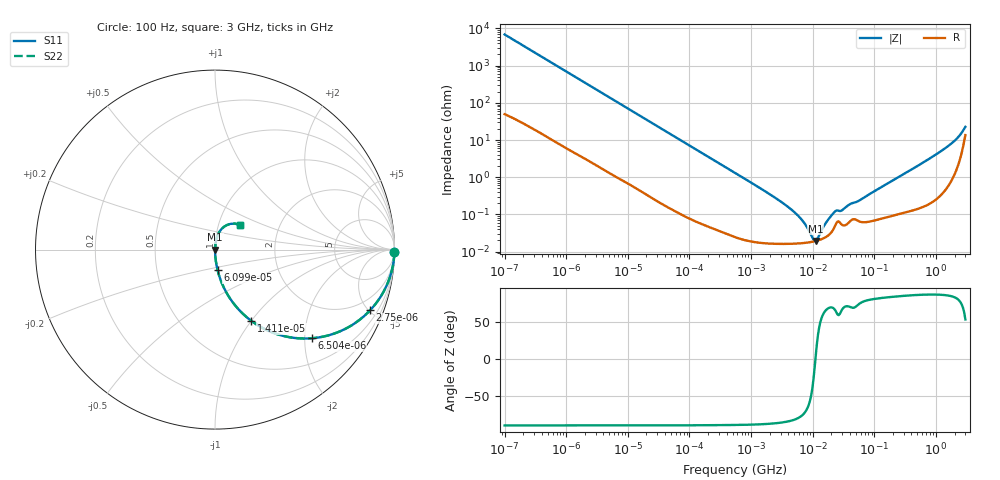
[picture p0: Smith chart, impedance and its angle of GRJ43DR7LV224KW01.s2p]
!Murata Part Number: GRJ43DR7LV224KW01
!These Parameters are Measured in Series Mode Connection
!Data Generated on Jun 19, 2026
!  o--ll--o
!Port1  Port2
!  o------o
!Operation Temp=25[degC], DC Bias Voltage=0[V]
!Freq. Start=100[Hz] Stop=3[GHz] 401[Steps]
# Hz S RI R 50
!Freq.(Hz) S11(Real) S11(Imag) S21(Real) S21(Imag) S12(Real) S12(Imag) S22(Real) S22(Imag)
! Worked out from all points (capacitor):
!   401 points, 100 Hz to 3 GHz, reference 50 ohm
!   read as one part in series: C = 232 nF near 109 Hz
!   lowest |Z| = 19.3 mohm at 11.14 MHz (marker M1)
!   series resonance near 11.06 MHz, so ESL is about 890 pH
!   S11 on the Smith chart (normalised r, x): 100 Hz: open; 2.75 kHz: 1.05, -5.08; 6.504 kHz: 1.02, -2.16; 14.12 kHz: 1.01, -1.00; 60.99 kHz: 1.00, -0.23; 3 GHz: 1.27, +0.36
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100  0.9997 -0.0146  0.000317 0.0146  0.000317 0.0146  0.9997 -0.0146
536  0.9934 -0.0768  0.00659 0.0768  0.00659 0.0768  0.9934 -0.0768
1788  0.9364 -0.2396  0.0636 0.2396  0.0636 0.2396  0.9364 -0.2396
2750  0.8637 -0.3385  0.1363 0.3385  0.1363 0.3385  0.8637 -0.3385
6504  0.5381 -0.4939  0.4619 0.4939  0.4619 0.4939  0.5381 -0.4939
14115  0.2024 -0.397  0.7976 0.397  0.7976 0.397  0.2024 -0.397
31977  0.0487 -0.2106  0.9513 0.2106  0.9513 0.2106  0.0487 -0.2106
60986  0.0146 -0.1149  0.9854 0.1149  0.9854 0.1149  0.0146 -0.1149
547723  0.000418 -0.0131  0.9996 0.0131  0.9996 0.0131  0.000418 -0.0131
2171352  0.000174 -0.0032  0.9998 0.0032  0.9998 0.0032  0.000174 -0.0032
4513443  0.000164 -0.00134  0.9998 0.00134  0.9998 0.00134  0.000164 -0.00134
6941223  0.00017 -0.000634  0.9998 0.000634  0.9998 0.000634  0.00017 -0.000634
9794414  0.000184 -0.00016  0.9998 0.00016  0.9998 0.00016  0.000184 -0.00016
1.11444e7  0.000193 1.02e-05  0.9998 -1.02e-05  0.9998 -1.02e-05  0.000193 1.02e-05
1.214626e7  0.0002 0.000124  0.9998 -0.000124  0.9998 -0.000124  0.0002 0.000124
1.713898e7  0.000259 0.000612  0.9997 -0.000612  0.9997 -0.000612  0.000259 0.000612
2.316512e7  0.000505 0.0011  0.9995 -0.0011  0.9995 -0.0011  0.000505 0.0011
2.999103e7  0.000522 0.00119  0.9995 -0.00119  0.9995 -0.00119  0.000522 0.00119
1.751444e8  0.000926 0.00717  0.9991 -0.00717  0.9991 -0.00717  0.000926 0.00717
1.324213e9  0.00698 0.0552  0.993 -0.0552  0.993 -0.0552  0.00698 0.0552
2.219584e9  0.0295 0.1062  0.9705 -0.1062  0.9705 -0.1062  0.0295 0.1062
3e9  0.1415 0.1368  0.8585 -0.1368  0.8585 -0.1368  0.1415 0.1368
